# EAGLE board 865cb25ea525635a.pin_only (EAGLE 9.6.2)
REV: A

Size 50.8 x 22.86 mm. Coordinates in mm from the lower left corner, seen from the top.
Outline: 2.54,0 48.26,0 arc90 50.8,2.54 50.8,20.32 arc90 48.26,22.86 2.54,22.86 arc90 0,20.32 0,2.54 arc90 2.54,0
Copper layers (1*16): Top 0.035mm / dielectric 1.5mm / Bottom 0.035mm
Design rules "adafruit 7-7 *": minimum track width 7mil, minimum drill 15.5mil, track to track 8mil, track to pad 7mil, pad to pad 7mil, via to via 7mil, smd to smd 7mil, copper to edge 10mil, drill to drill 8mil, minimum pad ring 10mil, minimum via ring 8mil, stop-mask expansion 2mil, vias tented up to drill 20mil, thermal gap 10mil
Net classes: 1 power: width 0.305 mm; 2 gnd: width 0.254 mm
Holes 2.54 mm at 48.26,20.32 48.26,2.54

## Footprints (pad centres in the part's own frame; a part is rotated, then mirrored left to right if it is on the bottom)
0805-NO = smd 1.24 x 1.5: 1 -0.95,0; 2 0.95,0
0603-NO = smd 1.075 x 1: 1 -0.85,0; 2 0.85,0
CHIPLED_0603_NOOUTLINE = smd 0.8 x 0.8: A 0,-0.75; C 0,0.75
JST_SH4 = smd 0.6 x 1.55: 1 -1.5,2.514; 2 -0.5,2.514; 3 0.5,2.514; 4 1.5,2.514 | smd 1.2 x 1.8: MT1 -2.8,-1.386; MT2 2.8,-1.386
SOD-123 = smd 1.4 x 1.4: A 1.85,0; C -1.85,0
B1,27 = smd 1.27 x 1.27: TP 0,0
QFN56_7MM_REDUCEDEPAD = smd 0.875 x 0.2: 1 -3.45,2.6; 2 -3.45,2.2; 3 -3.45,1.8; 4 -3.45,1.4; 5 -3.45,1; 6 -3.45,0.6; 7 -3.45,0.2; 8 -3.45,-0.2; 9 -3.45,-0.6; 10 -3.45,-1; 11 -3.45,-1.4; 12 -3.45,-1.8; 13 -3.45,-2.2; 14 -3.45,-2.6; 29 3.45,-2.6; 30 3.45,-2.2; 31 3.45,-1.8; 32 3.45,-1.4; 33 3.45,-1; 34 3.45,-0.6; 35 3.45,-0.2; 36 3.45,0.2; 37 3.45,0.6; 38 3.45,1; 39 3.45,1.4; 40 3.45,1.8; 41 3.45,2.2; 42 3.45,2.6 | smd 0.2 x 0.875: 15 -2.6,-3.45; 16 -2.2,-3.45; 17 -1.8,-3.45; 18 -1.4,-3.45; 19 -1,-3.45; 20 -0.6,-3.45; 21 -0.2,-3.45; 22 0.2,-3.45; 23 0.6,-3.45; 24 1,-3.45; 25 1.4,-3.45; 26 1.8,-3.45; 27 2.2,-3.45; 28 2.6,-3.45; 43 2.6,3.45; 44 2.2,3.45; 45 1.8,3.45; 46 1.4,3.45; 47 1,3.45; 48 0.6,3.45; 49 0.2,3.45; 50 -0.2,3.45; 51 -0.6,3.45; 52 -1,3.45; 53 -1.4,3.45; 54 -1.8,3.45; 55 -2.2,3.45; 56 -2.6,3.45 | smd 3.2 x 3.2: P$1 0,0
1X16_ROUND = drill 1 pad 1.676: 1 -19.05,0; 2 -16.51,0; 3 -13.97,0; 4 -11.43,0; 5 -8.89,0; 6 -6.35,0; 7 -3.81,0; 8 -1.27,0; 9 1.27,0; 10 3.81,0; 11 6.35,0; 12 8.89,0; 13 11.43,0; 14 13.97,0; 15 16.51,0; 16 19.05,0
1X12_ROUND = drill 1 pad 1.676: 1 -13.97,0; 2 -11.43,0; 3 -8.89,0; 4 -6.35,0; 5 -3.81,0; 6 -1.27,0; 7 1.27,0; 8 3.81,0; 9 6.35,0; 10 8.89,0; 11 11.43,0; 12 13.97,0
LED3535 = smd 1 x 0.85: 1 -1.75,0.875; 2 -1.75,-0.875; 3 1.75,-0.875; 4 1.75,0.875
SOT23-R = smd 0.635 x 1.016: 1 -0.95,-1; 2 0.95,-1; 3 0,1
BTN_KMR2_4.6X2.8 = smd 0.9 x 0.9: A 2.05,0.8; A' -2.05,0.8; B 2.05,-0.8; B' -2.05,-0.8
SOIC8_208MIL = smd 0.6 x 2.2: 1 -1.905,-3.315; 2 -0.635,-3.315; 3 0.635,-3.315; 4 1.905,-3.315; 5 1.905,3.315; 6 0.635,3.315; 7 -0.635,3.315; 8 -1.905,3.315
SOT23-5@1 = smd 0.55 x 1.2: 1 -0.95,-1.3; 2 0,-1.3; 3 0.95,-1.3; 4 0.95,1.3; 5 -0.95,1.3
SOT23-5 = smd 0.55 x 1.2: 1 -0.95,-1.3; 2 0,-1.3; 3 0.95,-1.3; 4 0.95,1.3; 5 -0.95,1.3
MOUNTINGHOLE_2.5_PLATED = drill 2.5 pad 3.2: P$1 0,0
FIDUCIAL_1MM = smd 1 x 1: 1 0,0
JSTPH2_BATT = smd 1 x 4.6: 1 -1,-3.7; 2 1,-3.7 | smd 1.6 x 3.4: NC1 -3.4,1.5; NC2 3.4,1.5
2X05_1.27MM_BOX_POSTS = smd 0.76 x 2.6: 1 -2.54,-2.15; 2 -2.54,2.15; 3 -1.27,-2.15; 4 -1.27,2.15; 5 0,-2.15; 6 0,2.15; 7 1.27,-2.15; 8 1.27,2.15; 9 2.54,-2.15; 10 2.54,2.15 | hole 1: -1.905,0; 1.905,0
USB_C_CUSB31-CFM2AX-01-X = smd 0.575 x 1.15: A1B12 -3.2,3.545; A4B9 -2.4,3.545; B1A12 3.2,3.545; B4A9 2.4,3.545 | smd 0.275 x 1.15: A5 -1.25,3.545; A6 -0.25,3.545; A7 0.25,3.545; A8 1.25,3.545; B5 1.75,3.545; B6 0.75,3.545; B7 -0.75,3.545; B8 -1.75,3.545 | drill 0.6 pad 1 long: M1 -4.32,2.97; M2 4.32,2.97; M3 -4.32,-1.21; M4 4.32,-1.21 | hole 0.65: 2.89,2.47; -2.89,2.47
CRYSTAL_2.5X2 = smd 0.9 x 0.75: 1 -0.825,-0.625; 2 0.825,-0.625; 3 0.825,0.625; 4 -0.825,0.625

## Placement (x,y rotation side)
C1  10µF  [0805-NO]  13.95,9.65 270 top
C2  22pF  [0603-NO]  28.26,18.41 0 top
C3  22pF  [0603-NO]  26.48,16.13 270 top
C4  10µF  [0805-NO]  15.05,13.89 180 top
C5  10uF  [0805-NO]  44.01,7.8 270 top
C6  0.1uF  [0603-NO]  27.88,9.53 90 top
C7  0.1uF  [0603-NO]  39.37,7.68 90 top
C8  1uF  [0603-NO]  40.89,7.68 270 top
C9  0.1uF  [0603-NO]  25.08,18.4 0 top
C10  1uF  [0603-NO]  38.35,5.28 0 top
C11  0.1uF  [0603-NO]  15.11,6.41 90 top
C12  0.1uF  [0603-NO]  27.37,12.89 90 top
C13  0.1uF  [0603-NO]  32.45,5.71 180 top
C14  0.1uF  [0603-NO]  33.97,17.65 0 top
C15  0.1uF  [0603-NO]  37.78,17.46 180 top
C16  0.1uF  [0603-NO]  42.42,7.68 270 top
C17  1uF  [0603-NO]  27.62,5.02 0 top
C20  10µF  [0805-NO]  15.88,17.21 270 top
CHG  ORANGE  [CHIPLED_0603_NOOUTLINE]  1.78,5.4 270 top
CONN1  STEMMA_I2C_QT  [JST_SH4]  48.26,8.26 90 top
D4  MBR540  [SOD-123]  12,12.19 180 top
D+1  TPB1,27  [B1,27]  1.46,10.22 0 bottom
D-1  TPB1,27  [B1,27]  1.4,12.83 0 bottom
IC1  RP2040_QFN56  [QFN56_7MM_REDUCEDEPAD]  34.42,11.43 270 top
JP1  [1X16_ROUND]  25.4,1.27 180 top
JP3  [1X12_ROUND]  30.48,21.65 0 top
L  RED  [CHIPLED_0603_NOOUTLINE]  1.82,17.42 90 top
LED1  WS2812B3535  [LED3535]  17.75,5.98 270 top
Q3  DMG341  [SOT23-R]  11.37,9.78 0 top
R1  10K  [0603-NO]  14.35,4.13 180 top
R2  10K  [0603-NO]  5.77,4.51 0 top
R3  10K  [0603-NO]  18.96,11.37 90 top
R4  10K  [0603-NO]  21.84,18.41 180 top
R5  10K  [0603-NO]  45.64,13.26 270 top
R6  1K  [0603-NO]  28.64,12.89 270 top
R7  10K  [0603-NO]  5.69,20.9 270 top
R8  5.1K  [0603-NO]  18.35,18.41 0 top
R9  27  [0603-NO]  7.68,12.32 90 top
R10  27  [0603-NO]  8.38,9.27 90 top
R11  1K  [0603-NO]  45.66,16.26 90 top
R12  5.1K  [0603-NO]  8.06,6.1 90 top
R13  5.1K  [0603-NO]  5.65,17.91 270 top
SW1  KMR2  [BTN_KMR2_4.6X2.8]  11.81,6.41 180 top
SW2  KMR2  [BTN_KMR2_4.6X2.8]  48.9,15.24 90 top
U1  2MB Flash  [SOIC8_208MIL]  42.42,14.73 180 top
U2  AP2112-3.3  [SOT23-5@1]  16.51,10.99 0 top
U3  MCP73831T-2ACI/OT  [SOT23-5]  18.54,15.53 0 top
U$9  [FEATHERLOGO]  35.24,5.97 0 bottom
U$12  [ADAFRUIT_3.5MM]  3.05,13.34 180 bottom
U$13  [PCBFEAT-REV-040]  3.49,17.08 0 bottom
U$28  [ADAFRUIT_3.5MM]  34.04,15.43 0 top
U$31  MOUNTINGHOLE2.5  [MOUNTINGHOLE_2.5_PLATED]  2.54,20.32 270 top
U$32  MOUNTINGHOLE2.5  [MOUNTINGHOLE_2.5_PLATED]  2.54,2.54 270 top
U$34  FIDUCIAL_1MM  [FIDUCIAL_1MM]  10.79,20.45 270 top
U$35  FIDUCIAL_1MM  [FIDUCIAL_1MM]  46.4,0.77 270 top
X1  JSTPH  [JSTPH2_BATT]  10.92,19.3 0 top
X2  [2X05_1.27MM_BOX_POSTS]  23.18,10.29 270 top
X6  USB Type C  [USB_C_CUSB31-CFM2AX-01-X]  2.6,11.43 270 top
Y1  12MHZ  [CRYSTAL_2.5X2]  28.32,16.19 270 top

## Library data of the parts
C1-C3 C5-C17 C20 CHG CONN1 D4 JP1 JP3 L LED1 Q3 R1-R13 SW1 SW2 U1-U3 U$9 U$12 U$28 X1 X2 X6 Y1 = microbuilder
C4 = microbuilder; COMPANY: ADAFRUIT INDUSTRIES; DRAWN: KTOWN; REV: A
D+1 D-1 = testpad
IC1 = adafruit_micro
U$13 = microbuilder; REV: A
U$31 U$32 U$34 U$35 = microbuilder; BOM: EXCLUDE

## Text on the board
tPlace: BAT | En | USB | 13 | 12 | 11 | 10 | 9 | 6 | 5 | SCL | SDA | 13 | USBBOOT | CHG | Neo | SWD | I2C | Reset | SCK | MOSI | MISO | RST | 3V | GND | A0 | A1 | A2 | A3 | 24 | 25 | RX | TX | D4
bPlace: 3.7/4.2V / LiPoly Batt / µUSB charge | 9 | 6 | 5 | SCL | BAT | En | USB | 13 | 12 | 11 | 10 | SDA | Feather / Pico 2040 | RST | 3V | 3V | GND | SCK | MOSI | MISO | A0 | A1 | A2 | A3 | A4 | A5 | RX | TX | D4

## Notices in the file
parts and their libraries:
microbuilder: This work is placed in the public domain, and may be freely used for commercial and non-commercial work with the following conditions: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
